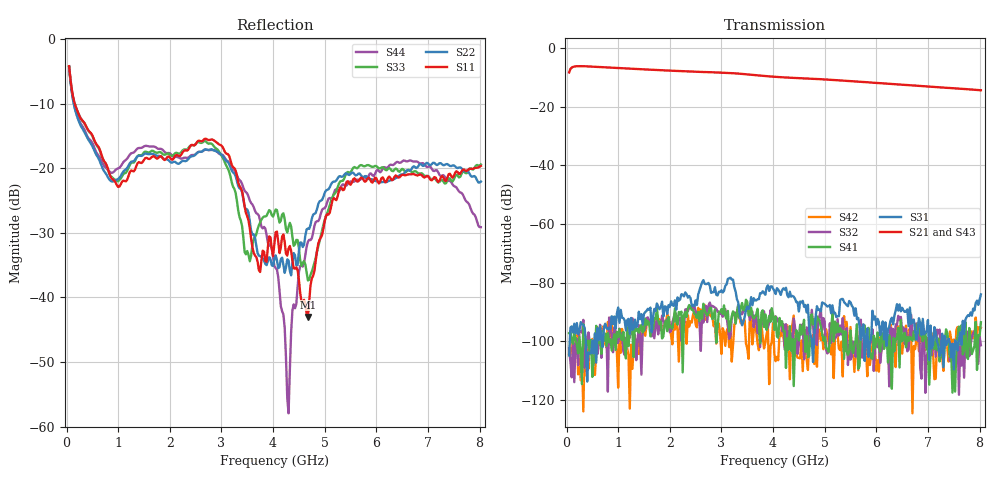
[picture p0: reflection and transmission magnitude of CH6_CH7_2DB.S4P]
!Agilent Technologies,E5071C,MY46316741,A.11.02
!Date: Mon Jun 01 10:33:59 2026
!Data & Calibration Information:
!1:CH6 INPUT 2:CH6 OUTPUT 3:CH7 INPUT 4:CH7 OUTPUT
!Freq	S11:SOLT4(ON)	S12:SOLT4(ON)	S13:SOLT4(ON)	S14:SOLT4(ON)
!	S21:SOLT4(ON)	S22:SOLT4(ON)	S23:SOLT4(ON)	S24:SOLT4(ON)
!	S31:SOLT4(ON)	S32:SOLT4(ON)	S33:SOLT4(ON)	S34:SOLT4(ON)
!	S41:SOLT4(ON)	S42:SOLT4(ON)	S43:SOLT4(ON)	S44:SOLT4(ON)
!PortZ  Port1:50+j0  Port2:50+j0  Port3:50+j0  Port4:50+j0
!Above PortZ is port z conversion or system Z0 setting when saving the data.
!When reading, reference impedance value at option line is always used.
# Hz S dB R 50
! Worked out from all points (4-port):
!   320 points, 50 MHz to 8.025 GHz, reference 50 ohm
!   strongest paths, dB at 50 MHz, 2.05 GHz, 4.05 GHz, 6.05 GHz, 8.025 GHz:
!     S21: -8.3, -7.7, -9.8, -11.9, -14.4
!     S43: -8.3, -7.7, -9.9, -12.0, -14.4
!     S31: -104.7, -87.6, -83.8, -93.4, -84.0
!     S41: -97.2, -95.6, -91.6, -101.4, -93.4
!     S32: -102.4, -93.5, -91.5, -100.9, -101.3
!     S42: -104.3, -101.0, -106.7, -110.3, -95.3
!   lowest |S11| = -43.0 dB at 4.675 GHz (marker M1), VSWR 1.01, Z = 49.4 - j0.38 ohm
!   |S11| at or under -10 dB: 160.2 MHz to end of sweep
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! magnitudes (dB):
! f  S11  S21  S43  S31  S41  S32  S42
! 50 MHz  -4.2  -8.3  -8.3  -104.7  -97.2  -102.4  -104.3
! 3.275 GHz  -20.3  -8.6  -8.7  -83.0  -94.0  -90.2  -93.4
! 4.075 GHz  -29.8  -9.9  -9.9  -81.9  -98.3  -92.1  -105.3
! 4.3 GHz  -32.4  -10.1  -10.1  -84.9  -102.8  -96.7  -97.8
! 4.675 GHz  -43.0  -10.4  -10.5  -87.5  -105.5  -95.6  -109.7
! 5.425 GHz  -22.1  -11.2  -11.2  -87.6  -103.2  -95.4  -93.3
! 8.025 GHz  -19.6  -14.4  -14.4  -84.0  -93.4  -101.3  -95.3
